FUNCTION_BLOCK ApplicationSubstate IMPLEMENTS I_ApplicationState;
VAR
	nullSubstate : NullSubstate;
	initialSubstate : I_Substate;
	_currentState : I_Substate;
END_VAR

METHOD PUBLIC AddSubstate
VAR_INPUT
	Substate : I_Substate;
END_VAR
VAR
	currentSubstate : I_Substate;
END_VAR
IF initialSubstate = 0 THEN
	initialSubstate := Substate;
	_currentState := Substate;
	RETURN;
END_IF

currentSubstate := initialSubstate;

WHILE currentSubstate.Next <> 0 DO
	currentSubstate := currentSubstate.Next;
END_WHILE

currentSubstate.Next := Substate;
END_METHOD

PROPERTY PUBLIC CurrentState : I_Substate
GET
IF _currentState = 0 THEN
	CurrentState := NullSubstate;
	RETURN;
END_IF

CurrentState := _currentState;
END_GET
END_PROPERTY

METHOD PUBLIC MoveNext : BOOL
VAR_INPUT
END_VAR
IF _currentState.Next = 0 THEN
	RETURN;
END_IF

_currentState := _currentState.Next;
MoveNext := TRUE;
END_METHOD

METHOD PUBLIC Reset
VAR_INPUT
END_VAR
_currentState := initialSubstate;
END_METHOD

END_FUNCTION_BLOCK
